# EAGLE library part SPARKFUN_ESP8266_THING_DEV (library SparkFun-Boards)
SparkFun Thing -Dev Board The SparkFun ESP8266 Thing Dev is a breakout and development board for the ESP8266 WiFi SoC, with an integrated FTDI USB-to-Serial chip. SparkFun Products: SparkFun ESP8266 Thing-Dev Board
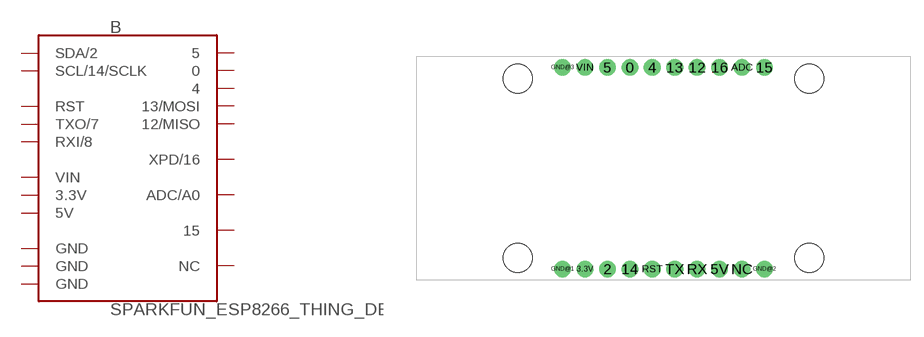
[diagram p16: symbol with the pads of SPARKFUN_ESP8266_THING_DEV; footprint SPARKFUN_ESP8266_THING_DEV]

Designator prefix B

## SPARKFUN_ESP8266_THING_DEV (SF_ID: WRL-13711)  [SPARKFUN_ESP8266_THING_DEV]
0  0
2  SDA/2
3.3V  3.3V  pwr
4  4
5  5
5V  5V  pwr
12  12/MISO
13  13/MOSI
14  SCL/14/SCLK
15  15
16  XPD/16
ADC  ADC/A0
GND@1  GND  pwr
GND@2  GND  pwr
GND@3  GND  pwr
NC  NC  nc
RST  RST  in
RX  RXI/8  in
TX  TXO/7  out
VIN  VIN  pwr

## Footprint SPARKFUN_ESP8266_THING_DEV (pad centres in mm)
SparkFun Thing Development Board Footprint Specifications: Pin count: 20 Pin pitch:0.1 inch Area: 2.2 x 1.0 inchees Example device(s): SparkFun Thing Development Board
drill 1.016 pad 1.88: 0 -2.54,11.43; 2 -5.08,-11.43; 3.3V -7.62,-11.43; 4 0,11.43; 5 -5.08,11.43; 5V 7.62,-11.43; 12 5.08,11.43; 13 2.54,11.43; 14 -2.54,-11.43; 15 12.7,11.43; 16 7.62,11.43; ADC 10.16,11.43; GND@1 -10.16,-11.43; GND@2 12.7,-11.43; GND@3 -10.16,11.43; NC 10.16,-11.43; RST 0,-11.43; RX 5.08,-11.43; TX 2.54,-11.43; VIN -7.62,11.43
hole 3.302 at -15.24,-10.16
hole 3.302 at -15.24,10.16
hole 3.302 at 17.78,10.16
hole 3.302 at 17.78,-10.16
